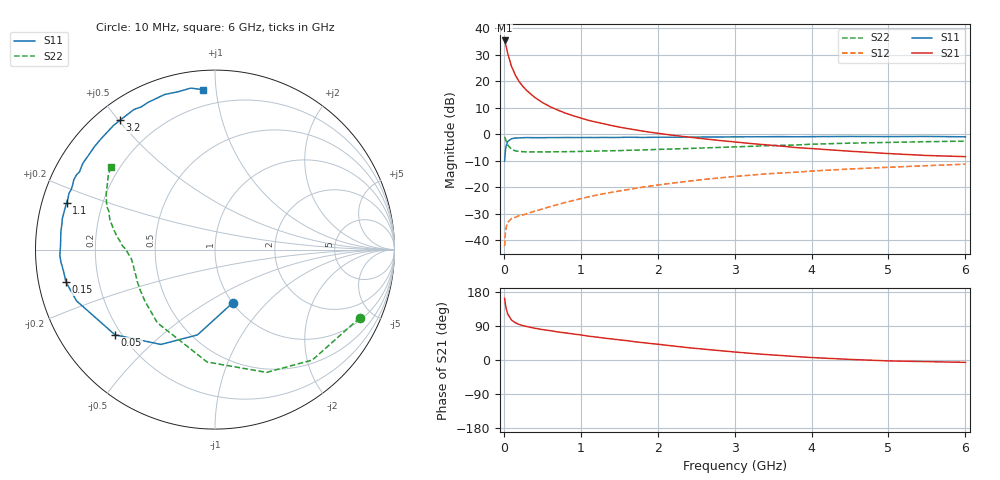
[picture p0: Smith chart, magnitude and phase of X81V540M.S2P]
! SIEMENS Small Signal Semiconductors
! BFP136W
! Si NPN RF Bipolar Junction Transistor in SOT343
! VCE = 1.5 V  IC = 40 mA
! Common Emitter S-Parameters:  September  1994
# GHz  S  MA  R  50
!  f  S11  S21  S12  S22
! GHz  MAG  ANG  MAG  ANG  MAG  ANG  MAG  ANG
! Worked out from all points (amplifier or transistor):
!   40 points, 10 MHz to 6 GHz, reference 50 ohm
!   highest |S21| = 35.4 dB at 10 MHz (marker M1)
!   |S21| within 3 dB of that: start of sweep to 35.54 MHz
!   unconditionally stable (mu >= 1): 643 MHz to 2.888 GHz
!   at 200 MHz: K = 0.50, MSG = 25.3 dB, |S12| = -30.7 dB
!   at 1.5 GHz: K = 1.14, MAG = 9.8 dB, |S12| = -21.4 dB
!   at 6 GHz: K = 0.99, MSG = 1.4 dB, |S12| = -11.3 dB
!   S11 on the Smith chart (normalised r, x): 10 MHz: 1.01, -0.66; 50 MHz: 0.17, -0.36; 150 MHz: 0.08, -0.11; 1.1 GHz: 0.07, +0.15; 3.2 GHz: 0.07, +0.51; 6 GHz: 0.10, +0.92
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0.01  0.3115 -71.2  59.06 162.7  0.0077 72.1  0.8914 -25.3
0.02  0.485 -101.6  52.26 147.8  0.0135 60.4  0.8202 -48.6
0.03  0.6084 -119.7  45.45 136.4  0.0175 50.7  0.7421 -67.2
0.05  0.7322 -139.6  33.63 121.6  0.0216 38.1  0.6279 -94.0
0.1  0.8227 -159.7  19.07 105.4  0.0256 29.7  0.5193 -128.2
0.15  0.8499 -167.7  13.05 98.2  0.027 29.8  0.4847 -143.7
0.2  0.8527 -172.1  9.821 93.8  0.0291 30.6  0.4733 -152.2
0.25  0.861 -175.3  7.928 90.6  0.03 32.7  0.4683 -157.6
0.3  0.8653 -177.7  6.633 88.2  0.0316 35.3  0.4642 -161.2
0.4  0.8609 178.3  4.994 83.9  0.0352 39.6  0.4634 -165.9
0.5  0.862 175.4  3.983 80.3  0.0387 43.4  0.4637 -169.0
0.6  0.8645 173.3  3.323 77.5  0.043 46.3  0.4652 -171.0
0.7  0.8647 170.5  2.862 74.1  0.047 49.4  0.467 -172.2
0.9  0.867 166.9  2.241 68.7  0.0559 52.3  0.4713 -174.6
1.1  0.8675 162.4  1.833 62.9  0.0655 54.2  0.4779 -176.1
1.5  0.8708 155.7  1.365 53.3  0.0849 56.0  0.4913 -178.9
1.8  0.8704 150.1  1.15 46.0  0.0999 55.1  0.5051 178.8
2.2  0.879 143.3  0.956 37.0  0.1199 53.4  0.5263 175.8
3.2  0.8944 126.2  0.67 17.7  0.1684 45.5  0.5906 166.5
4.5  0.9086 108.0  0.478 1.6  0.2208 33.6  0.6793 153.3
5.5  0.9098 98.5  0.397 -4.3  0.2552 25.5  0.7243 145.2
6  0.8937 94.4  0.378 -6.2  0.272 21.1  0.7405 141.8
